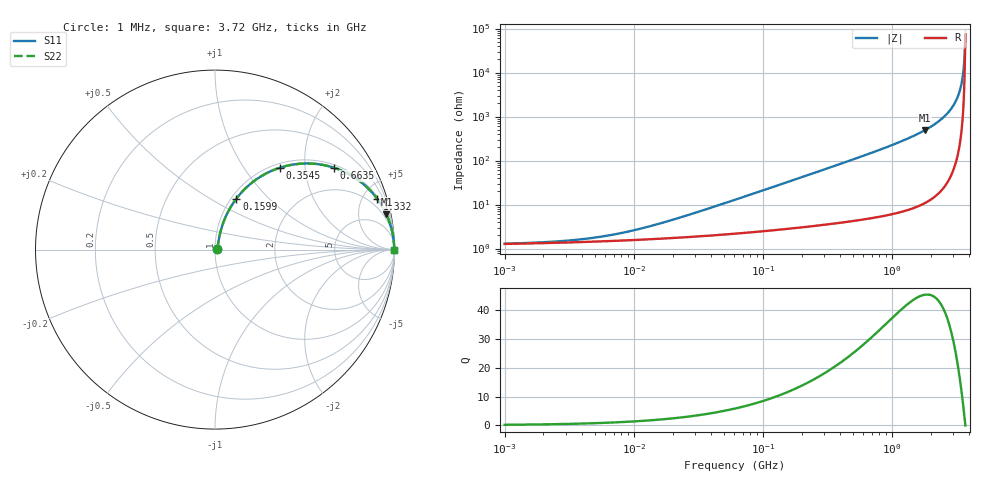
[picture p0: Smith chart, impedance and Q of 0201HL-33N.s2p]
# MHz  S  MA  R  50
!Freq  MagS11  AngS11  MagS21  AngS21  MagS12  AngS12  MagS22  AngS22
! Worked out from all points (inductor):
!   828 points, 1 MHz to 3.72 GHz, reference 50 ohm
!   read as one part in series: L = 33 nH near 26.41 MHz
!   highest Q = 45.4 at 1.795 GHz (marker M1), where L = 43 nH
!   self-resonance near 3.711 GHz
!   S11 on the Smith chart (normalised r, x): 1 MHz: 1.03, +0.00; 159.9 MHz: 1.06, +0.66; 354.5 MHz: 1.07, +1.48; 663.5 MHz: 1.10, +2.84; 1.332 GHz: 1.15, +6.33; 3.72 GHz: open
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1  0.01273 9.1  0.9874 -0.1  0.9874 -0.1  0.01273 9.1
3.947749  0.01602 29.8  0.9861 -0.5  0.9861 -0.5  0.01602 29.8
7.689208  0.02161 45.7  0.985 -0.9  0.985 -0.9  0.02161 45.7
15.58473  0.03573 60.9  0.9831 -1.8  0.9831 -1.8  0.03573 60.9
61.52459  0.1257 73.2  0.9711 -7.1  0.9711 -7.1  0.1257 73.2
159.9192  0.3085 67.2  0.9255 -17.9  0.9255 -17.9  0.3085 67.2
240.4789  0.4374 60.5  0.8717 -25.9  0.8717 -25.9  0.4374 60.5
354.4953  0.5826 51.6  0.7844 -35.6  0.7844 -35.6  0.5826 51.6
487.4101  0.7031 43.0  0.6832 -44.6  0.6832 -44.6  0.7031 43.0
663.5247  0.8053 34.5  0.5664 -53.6  0.5664 -53.6  0.8053 34.5
949.3504  0.8939 25.1  0.4244 -63.3  0.4244 -63.3  0.8939 25.1
1331.537  0.9472 17.4  0.299 -71.2  0.299 -71.2  0.9472 17.4
1794.711  0.9752 11.6  0.201 -77.1  0.201 -77.1  0.9752 11.6
2189.888  0.9867 8.2  0.1419 -80.6  0.1419 -80.6  0.9867 8.2
2567.816  0.9928 5.6  0.09756 -83.0  0.09756 -83.0  0.9928 5.6
2893.479  0.9958 3.8  0.06551 -84.5  0.06551 -84.5  0.9958 3.8
3164.556  0.9974 2.4  0.04195 -85.2  0.04195 -85.2  0.9974 2.4
3359.24  0.9981 1.5  0.02641 -85.0  0.02641 -85.0  0.9981 1.5
3495.638  0.9984 0.9  0.0161 -83.8  0.0161 -83.8  0.9984 0.9
3530.595  0.9984 0.8  0.01353 -83.0  0.01353 -83.0  0.9984 0.8
3710.691  0.9986 0.0  0.001473 -22.3  0.001473 -22.3  0.9986 0.0
3720  0.9986 -0.0  0.00136 3.8  0.00136 3.8  0.9986 -0.0
